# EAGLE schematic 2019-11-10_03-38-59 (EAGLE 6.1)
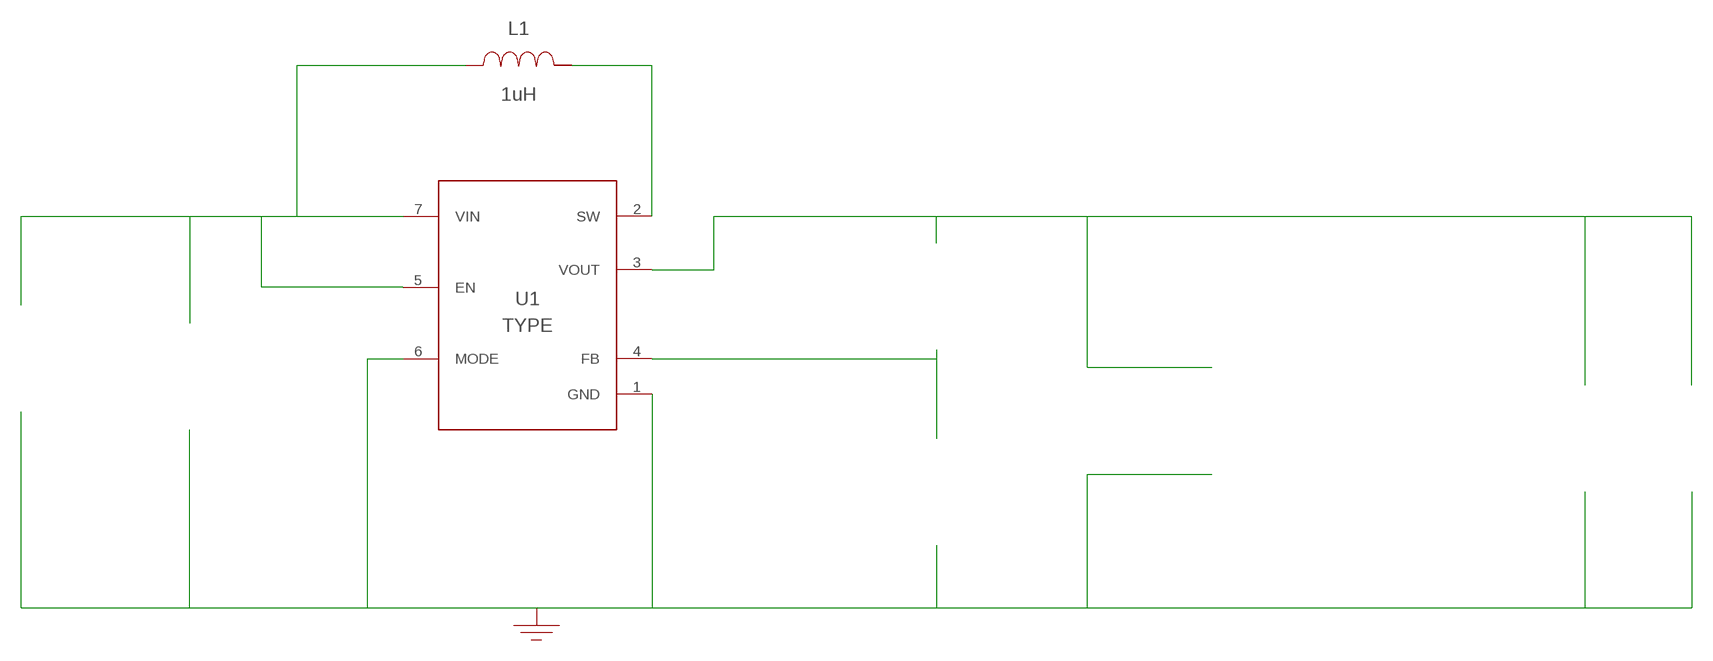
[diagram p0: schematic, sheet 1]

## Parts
CIN  10uF  C0805C106K8PACTUC0805C106K8PACTU  [0805]  (not placed on a sheet)
COUT  10uF  GRM21BR71A106KE51LGRM21BR71A106KE51L  [0805]  (not placed on a sheet)
COUT_2  10uF  GRM21BR71A106KE51LGRM21BR71A106KE51L  [0805]  (not placed on a sheet)
GND  WB_GND  WB_GNDWB_GND  [WB_GND]
IOUT  WB_PWL_CURRENT_LOAD  WB_PWL_CURRENT_LOADWB_PWL_CURRENT_LOAD  [WB_PWL_CURRENT_LOAD]  (not placed on a sheet)
L1  1uH  XFL4020-102MEBXFL4020-102MEB  [XFL4020]
RFBB  100k  CRCW0402100KFKEDCRCW0402100KFKED  [0402]  (not placed on a sheet)
RFBT  732k  CRCW0402732KFKEDCRCW0402732KFKED  [0402]  (not placed on a sheet)
RLOAD  WB_LOAD_RESISTOR  WB_LOAD_RESISTORWB_LOAD_RESISTOR  [WB_LOAD_RESISTOR]  (not placed on a sheet)
U1  TPS61022RWUR  TPS61022RWURTPS61022RWUR  [RWU0007A]
VIN  WB_BATTERY  WB_BATTERYWB_BATTERY  [WB_BATTERY]  (not placed on a sheet)

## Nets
0: Cin.2@2 Cout.2@2 Cout_2.2@2 GND.1 Iout.-@2 Rfbb.2@2 Rload.2@2 U1.1(GND) U1.6(MODE) Vin.-@2
2: Cin.1@1 L1.1 U1.5(EN) U1.7(VIN) Vin.+@1
3: Rfbb.1@1 Rfbt.2@2 U1.4(FB)
4: L1.2 U1.2(SW)
5: Cout.1@1 Cout_2.1@1 Iout.+@1 Rfbt.1@1 Rload.1@1 U1.3(VOUT)
Unconnected: CIN.1 CIN.2 COUT.1 COUT.2 COUT_2.1 COUT_2.2 IOUT.1(+) IOUT.2(-) RFBB.1 RFBB.2 RFBT.1 RFBT.2 RLOAD.1 RLOAD.2 VIN.1(+) VIN.2(-)

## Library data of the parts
CIN = AcceleratedDesigns_Lib:C0805C106K8PACTU; Cap: 1.0E-5; ESR: 0.0030; IRMS: 11.43; Manufacturer_Name: Kemet; Manufacturer_Part_Number: C0805C106K8PACTU; VDC: 10.0; Vendor: Kemet
COUT COUT_2 = AcceleratedDesigns_Lib:GRM21BR71A106KE51L; Cap: 1.0E-5; ESR: 0.0030; IRMS: 0.0; Manufacturer_Name: MuRata; Manufacturer_Part_Number: GRM21BR71A106KE51L; VDC: 10.0; Vendor: MuRata
GND = AcceleratedDesigns_Lib:WB_GND; Manufacturer_Name: WB_GND; Manufacturer_Part_Number: WB_GND; PowerPortType: POWER_GROUND; Value: Value
IOUT = AcceleratedDesigns_Lib:WB_PWL_CURRENT_LOAD; Manufacturer_Name: WB_PWL_CURRENT_LOAD; Manufacturer_Part_Number: WB_PWL_CURRENT_LOAD; PowerPortType: POWER_GROUND; Value: Value
L1 = AcceleratedDesigns_Lib:XFL4020-102MEB; DCR: 0.01; IDC: 5.4; L: 1.0E-6; Manufacturer_Name: Coilcraft; Manufacturer_Part_Number: XFL4020-102MEB; Vendor: Coilcraft
RFBB = AcceleratedDesigns_Lib:CRCW0402100KFKED; Manufacturer_Name: Vishay-Dale; Manufacturer_Part_Number: CRCW0402100KFKED; Power: 0.063; Resistance: 100000.0; Tolerance: 1.0; Vendor: Vishay-Dale
RFBT = AcceleratedDesigns_Lib:CRCW0402732KFKED; Manufacturer_Name: Vishay-Dale; Manufacturer_Part_Number: CRCW0402732KFKED; Power: 0.063; Resistance: 732000.0; Tolerance: 1.0; Vendor: Vishay-Dale
RLOAD = AcceleratedDesigns_Lib:WB_LOAD_RESISTOR; Manufacturer_Name: WB_LOAD_RESISTOR; Manufacturer_Part_Number: WB_LOAD_RESISTOR; PowerPortType: POWER_GROUND; Value: Value
U1 = AcceleratedDesigns_Lib:TPS61022RWUR; Manufacturer: Texas Instruments; Manufacturer_Name: Texas Instruments; Manufacturer_Part_Number: TPS61022RWUR; PartNumber: TPS61022RWUR; RefDes: RefDes; TYPE: TYPE; Value: Value
VIN = AcceleratedDesigns_Lib:WB_BATTERY; Manufacturer_Name: WB_BATTERY; Manufacturer_Part_Number: WB_BATTERY; PowerPortType: POWER_GROUND; Value: Value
